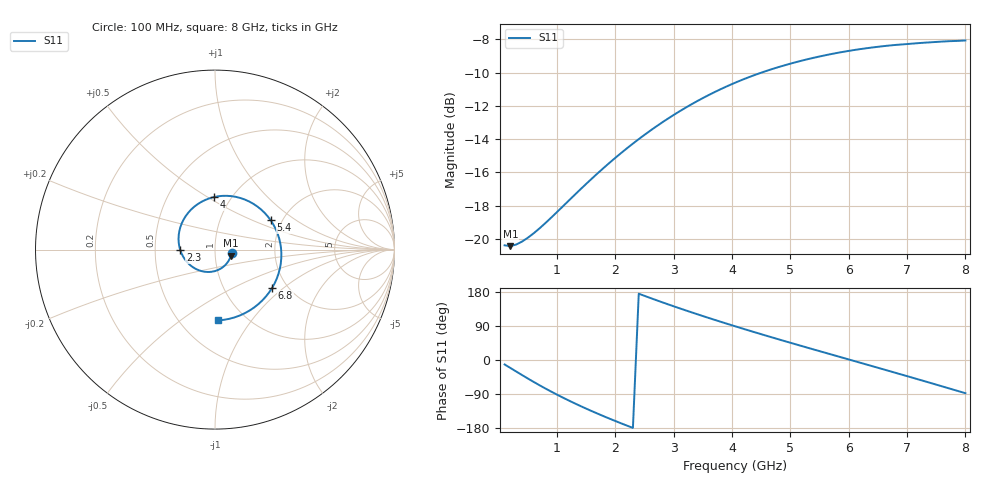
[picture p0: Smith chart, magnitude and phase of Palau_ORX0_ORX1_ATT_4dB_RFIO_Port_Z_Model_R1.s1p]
! Created Fri Oct  9 14:29:04 2020
! Palau ORX0/ORX1 RFIO Port Impedance Model.
! Attenuation  : 4 dB.
! Revision		: R1.
! Impedance Mode 	: Balanced Differential-Mode.
! Impedance Format 	: Series Equivalent Differential Impedance (SEDZ).
# hz S ma R 100
! 1 Port Network Data from SP1.SP block
! freq  magS11  angS11
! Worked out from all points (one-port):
!   80 points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, 100 MHz to 8 GHz, reference 100 ohm
!   lowest |S11| = -20.4 dB at 200 MHz (marker M1), VSWR 1.21, Z = 119 - j8.24 ohm
!   |S11| at or under -10 dB: start of sweep to 4.499 GHz
!   S11 on the Smith chart (normalised r, x): 100 MHz: 1.21, -0.05; 2.3 GHz: 0.68, -0.00; 4 GHz: 0.83, +0.53; 5.4 GHz: 1.75, +0.65; 6.8 GHz: 1.67, -0.84; 8 GHz: 0.75, -0.70
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1e8  0.09566 -11.8
2e8  0.0951 -21.1
4e8  0.09821 -39.8
7e8  0.1076 -66.7
1.1e9  0.1254 -99.3
1.3e9  0.1356 -114.2
1.6e9  0.1521 -135.2
2.1e9  0.1814 -167.2
2.3e9  0.1935 -179.2
2.7e9  0.2179 158.0
3.1e9  0.242 136.4
3.3e9  0.2538 126.0
3.6e9  0.2709 110.9
4e9  0.2924 91.5
4.1e9  0.2974 86.7
4.3e9  0.3071 77.3
4.6e9  0.3206 63.5
4.8e9  0.3289 54.4
5.1e9  0.3403 41.0
5.4e9  0.3507 27.8
5.8e9  0.3626 10.2
6.1e9  0.3702 -2.9
6.4e9  0.3765 -16.1
6.8e9  0.3832 -33.8
7.1e9  0.3869 -47.0
7.4e9  0.3903 -60.5
7.6e9  0.3923 -69.5
8e9  0.3953 -87.6
